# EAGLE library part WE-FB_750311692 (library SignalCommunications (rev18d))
WE-FB Flyback Transformer suitable for LT3573/ LT3574/ LT3575/ LT3748 Characteristics easy design in solution less external components needed small board space low cost no optocoupler needed! long term reliability voltage control no aging same external parts for different output voltages easy design of custom power supply due to standard circuit and change of transformers and two components for feedback loop Isolation voltage up to 2.5 kV Applications Isolated power design Sensor interfaces Isolated telecom converters Power over Ethernet Details see: http://katalog.we-online.de/en/pbs/WE-FB_Linear? Updated 2014-07-07 2014 (C) Wurth Elektronik
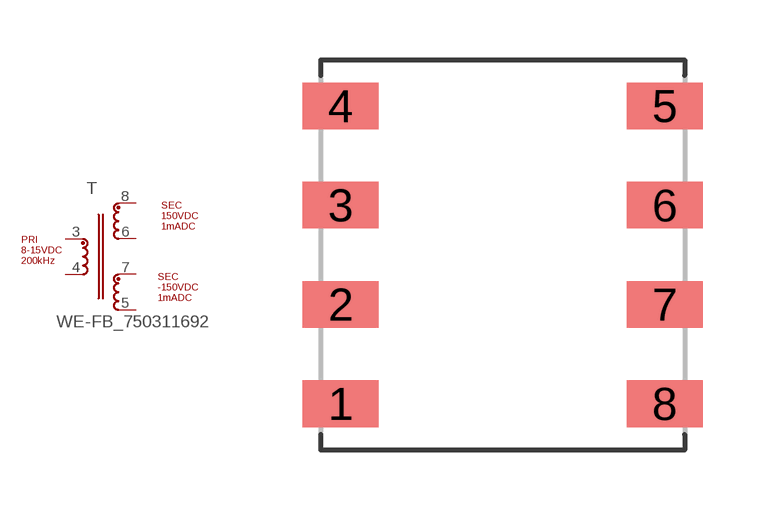
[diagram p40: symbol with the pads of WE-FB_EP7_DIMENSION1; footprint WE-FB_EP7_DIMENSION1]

Designator prefix T

## WE-FB_750311692  [WE-FB_EP7_DIMENSION1]
3  1  pas
4  6  pas
5  5  pas
6  3  pas
7  4  pas
8  2  pas

## Footprint WE-FB_EP7_DIMENSION1 (pad centres in mm)
Transformer, EP7* SMD 8Pin für WE-FB
smd 1.91 x 1.17: 1 -4.065,-3.735; 2 -4.065,-1.245; 3 -4.065,1.245; 4 -4.065,3.735; 5 4.065,3.735; 6 4.065,1.245; 7 4.065,-1.245; 8 4.065,-3.735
